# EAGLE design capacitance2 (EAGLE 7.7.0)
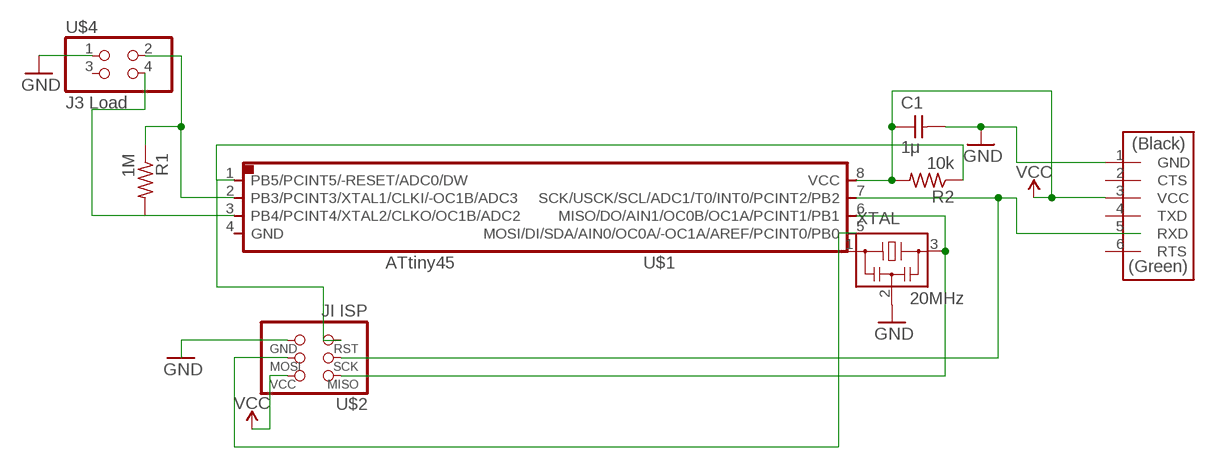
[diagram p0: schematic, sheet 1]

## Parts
C1  1μ  CAP-UNPOLARIZEDFAB  [C1206FAB]
R1  1M  RES-US1206FAB  [R1206FAB]
R2  10k  RES-US1206FAB  [R1206FAB]
U$1  ATTINY45SI  [SOIC8]
U$2  JI ISP  AVRISPSMD  [2X03SMD]
U$3  FTDI-SMD-HEADER  [1X06SMD]
U$4  J3 Load  PINHD-2X2-SMD  [2X02SMD]
XTAL  20MHz  RESONATOR  [EFOBM]

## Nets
GND: C1.2 U$2.6(GND) U$3.1(GND) U$4.1 XTAL.2
N$2: U$1.6(MISO/DO/AIN1/OC0B/OC1A/PCINT1/PB1) U$2.1(MISO) XTAL.3
N$4: R2.1 U$1.1(PB5/PCINT5/-RESET/ADC0/DW) U$2.5(RST)
N$5: R1.1 U$1.2(PB3/PCINT3/XTAL1/CLKI/-OC1B/ADC3) U$4.2
N$7: U$1.7(SCK/USCK/SCL/ADC1/T0/INT0/PCINT2/PB2) U$2.3(SCK)
N$8: R1.2 U$1.3(PB4/PCINT4/XTAL2/CLKO/OC1B/ADC2) U$4.4
N$12: U$1.5(MOSI/DI/SDA/AIN0/OC0A/-OC1A/AREF/PCINT0/PB0) U$2.4(MOSI) XTAL.1
VCC: C1.1 R2.2 U$1.8(VCC) U$2.2(VCC) U$3.3(VCC)
Unconnected: U$1.4(GND) U$3.2(CTS) U$3.4(TXD) U$3.5(RXD) U$3.6(RTS) U$4.3

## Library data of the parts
C1 = fab:CAP-UNPOLARIZED
R1 R2 = fab:RES-US: Resistor (US Symbol)
U$1 = fab:ATTINY45
U$2 = fab:AVRISP
U$3 = fab:FTDI-SMD-HEADER
U$4 = fab:PINHD-2X2-SMD
XTAL = fab:RESONATOR

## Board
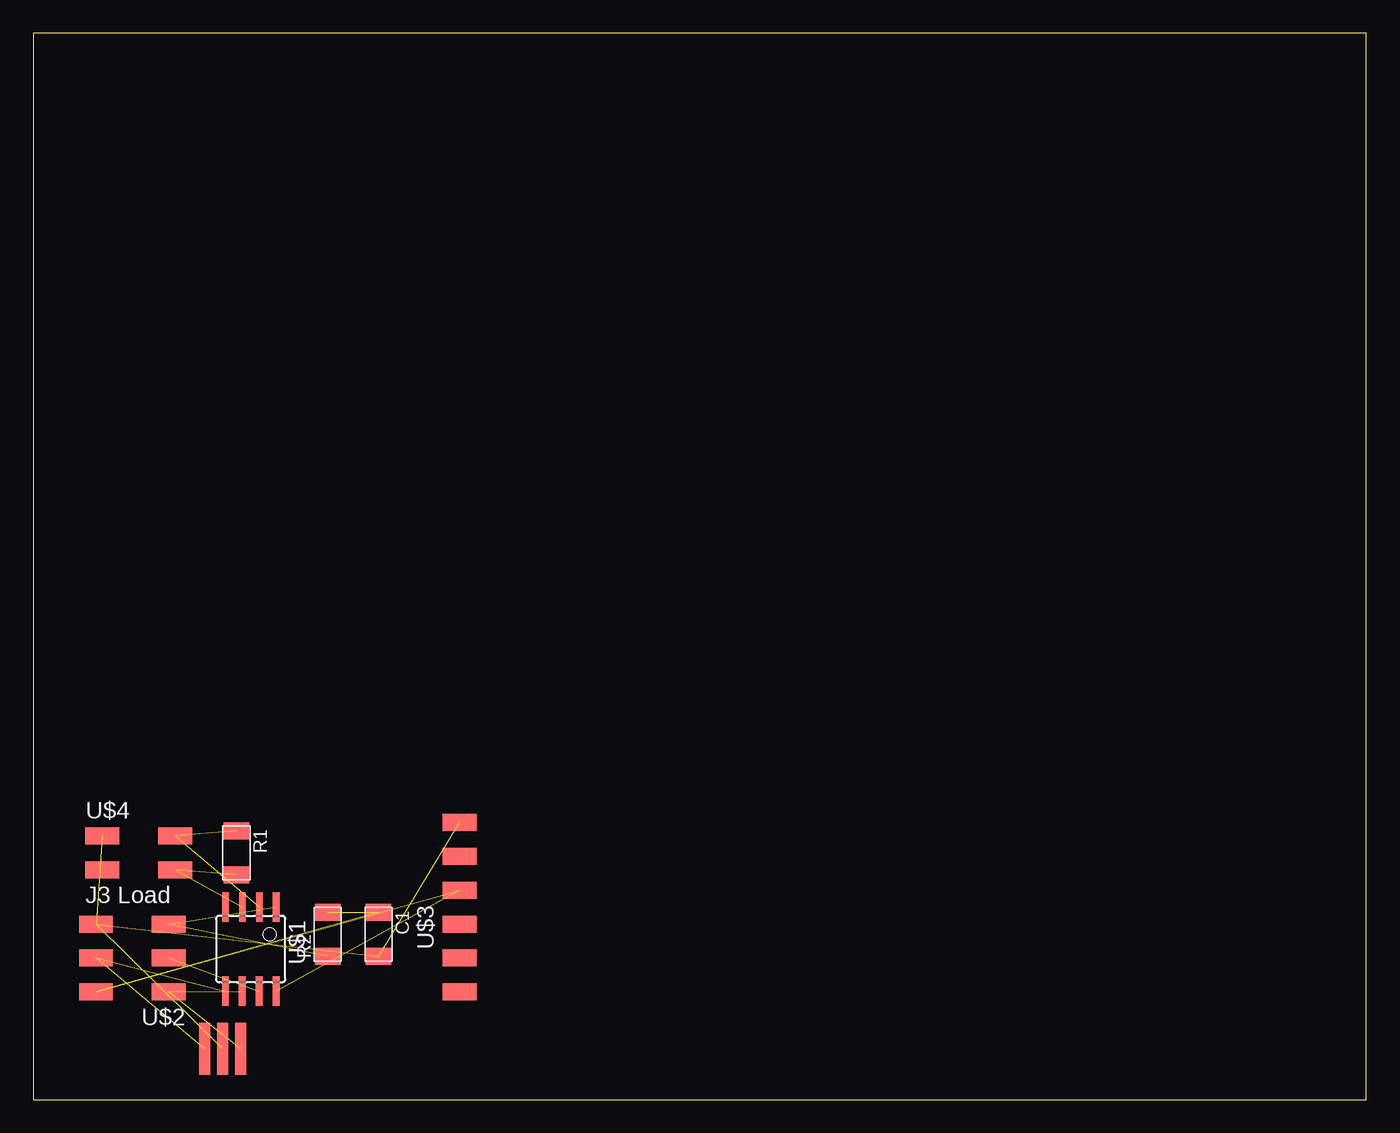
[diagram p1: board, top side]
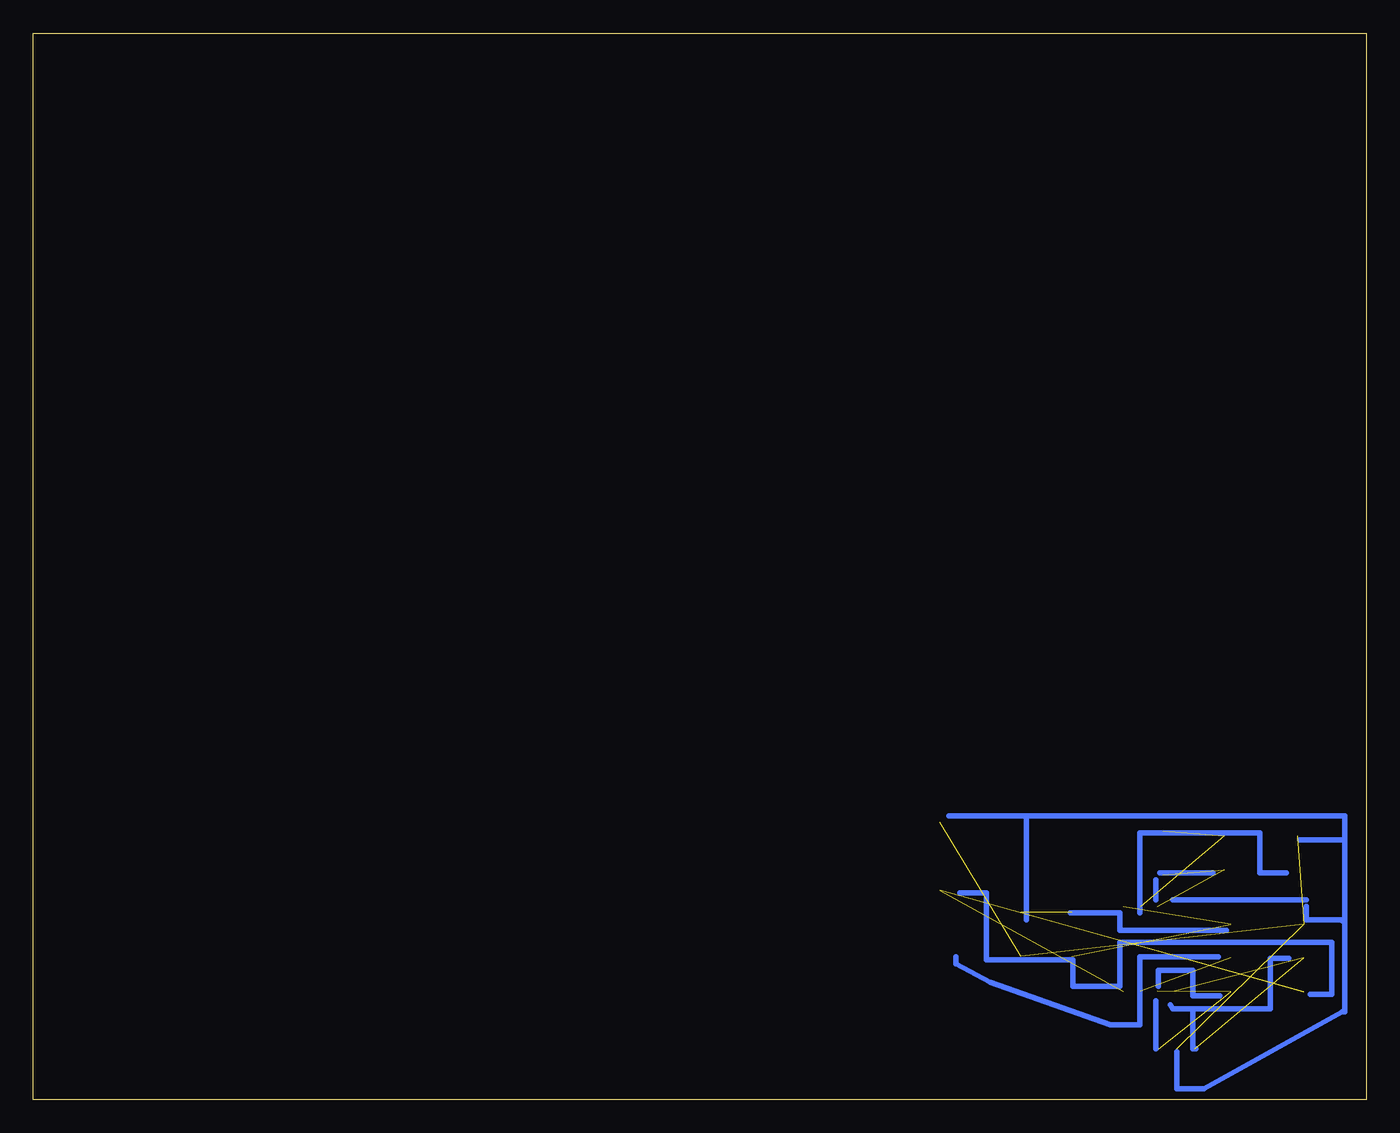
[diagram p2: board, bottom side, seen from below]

Size 100 x 80 mm. Coordinates in mm from the lower left corner, seen from the top.
Outline: 0,0 100,0 100,80 0,80 0,0
Copper layers (1*16): Top 0.035mm / dielectric 1.5mm / Bottom 0.035mm
Design rules "default": minimum track width 10mil, minimum drill 24mil, track to track 8mil, track to pad 8mil, pad to pad 8mil, via to via 8mil, smd to smd 8mil, copper to edge 40mil, drill to drill 8mil, minimum pad ring 10mil, minimum via ring 8mil, stop-mask expansion 4mil, vias tented up to drill 0mil, thermal gap 10mil

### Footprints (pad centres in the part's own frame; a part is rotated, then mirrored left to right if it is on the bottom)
C1206FAB = smd 1.27 x 1.905: 1 -1.651,0; 2 1.651,0
R1206FAB = smd 1.27 x 1.905: 1 -1.651,0; 2 1.651,0
SOIC8 = smd 0.5 x 2.2: 1 -1.905,-3.154; 2 -0.645,-3.154; 3 0.625,-3.154; 4 1.895,-3.154; 5 1.905,3.154; 6 0.635,3.154; 7 -0.635,3.154; 8 -1.905,3.154
2X03SMD = smd 2.54 x 1.27: 1 -2.54,2.54; 2 2.92,2.54; 3 -2.54,0; 4 2.92,0; 5 -2.54,-2.54; 6 2.92,-2.54
1X06SMD = smd 2.54 x 1.27: 1 0,6.35; 2 0,3.81; 3 0,1.27; 4 0,-1.27; 5 0,-3.81; 6 0,-6.35
2X02SMD = smd 2.54 x 1.27: 1 -2.54,1.27; 2 2.92,1.27; 3 -2.54,-1.27; 4 2.92,-1.27
EFOBM = smd 0.8 x 3.9: 1 -1.35,0; 2 0,0; 3 1.35,0

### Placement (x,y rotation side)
C1  25.9,12.39 270 top
R1  15.24,18.51 270 top
R2  22.09,12.39 90 top
U$1  16.31,11.29 180 top
U$2  7.62,10.62 180 top
U$3  31.98,14.43 0 top
U$4  7.72,18.51 0 top
XTAL  14.2,3.8 0 top

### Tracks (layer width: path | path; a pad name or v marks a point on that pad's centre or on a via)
GND  (4 unrouted)
N$1
  Bottom 0.406: 15.8,15 15.8,16.5
N$2  (2 unrouted)
N$3
  Bottom 0.406: 4.2,7.9 2.6,7.9 2.6,11.8 18.5,11.8 18.5,8.5 22,8.5 22,10.5 28.5,10.5 28.5,15.5 30.5,15.5
N$4  (2 unrouted)
N$5  (2 unrouted)
N$6
  Bottom 0.406: 15.8,7.4 15.8,3.8
N$7  (1 unrouted)
N$8  (2 unrouted)
N$9
  Bottom 0.406: 11.5,17 15.5,17
N$10
  Bottom 0.406: 10.5,12.7 18.5,12.7 18.5,14
N$11
  Bottom 0.406: 6,17 8,17 8,20 17,20 17,14
N$12  (2 unrouted)
N$13
  Bottom 0.406: 11.1,10.7 17,10.7 17,6
N$14
  Bottom 0.406: 12.8,3.8 13,3.8 13,6.6
N$15
  Bottom 0.406: 17,7 17,5.6 19.2,5.6 28.2,8.8 30.8,10.2 30.8,10.7
N$16
  Bottom 0.406: 14.7,7.1 14.5,6.8 7.2,6.8 7.2,10.6 5.8,10.6
N$17
  Bottom 0.406: 15.6,8.5 15.6,9.7 13,9.7 13,7.8 11,7.8
N$18
  Bottom 0.406: 14.5,15 4.5,15
N$19
  Bottom 0.406: 4.5,14.5 4.5,13.5 1.6,13.5 1.6,19.5 | 25.5,13.5 25.5,21.3 | 25.5,21.3 1.6,21.3 1.6,19.5 | 25.5,21.3 26.3,21.3 31.3,21.3 | 1.6,19.5 5,19.5
N$20
  Bottom 0.406: 1.8,13.4 1.6,13.4 1.6,6.6 1.8,6.6 12.2,0.8 14.2,0.8 14.2,3.6
N$21
  Bottom 0.406: 18.6,14 22.2,14
VCC  (4 unrouted)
